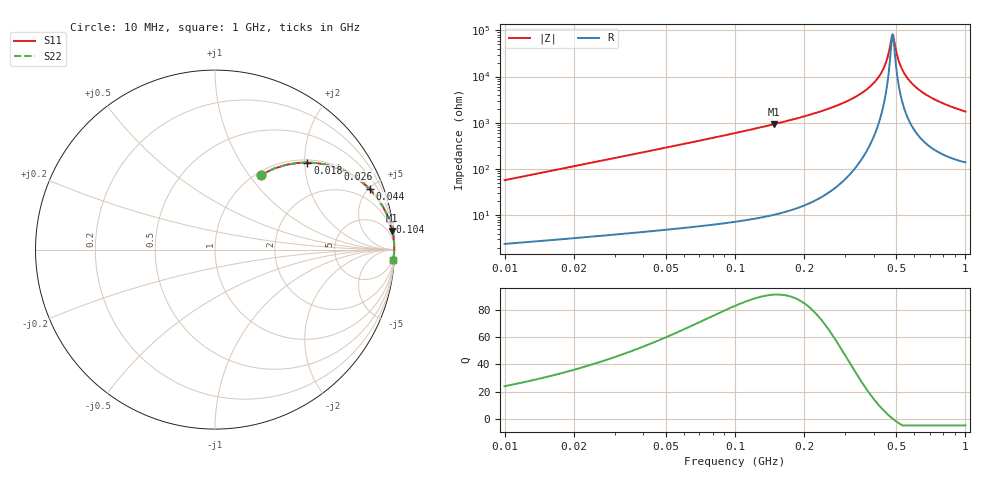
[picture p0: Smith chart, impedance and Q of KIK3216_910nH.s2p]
!version-2
!date-01.2022
!Series
# MHz S RI R 50
!Freq ReS11 ImS11 ReS21 ImS21 ReS12 ImS12 ReS22 ImS22
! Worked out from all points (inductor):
!   496 points, 10 MHz to 1 GHz, reference 50 ohm
!   read as one part in series: L = 910 nH near 14 MHz
!   highest Q = 91.3 at 148 MHz (marker M1), where L = 1 uH
!   self-resonance near 482 MHz
!   S11 on the Smith chart (normalised r, x): 10 MHz: 1.05, +1.14; 18 MHz: 1.06, +2.06; 26 MHz: 1.07, +2.98; 44 MHz: 1.09, +5.07; 104 MHz: 1, +12; 1 GHz: 4, -35
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10  0.2557 0.4158  0.7443 -0.4158  0.7443 -0.4158  0.2557 0.4158
18  0.5149 0.4852  0.4851 -0.4852  0.4851 -0.4852  0.5149 0.4852
26  0.6857 0.4524  0.3143 -0.4524  0.3143 -0.4524  0.6857 0.4524
44  0.8611 0.337  0.1389 -0.337  0.1389 -0.337  0.8611 0.337
66  0.9336 0.2418  0.0664 -0.2418  0.0664 -0.2418  0.9336 0.2418
104  0.9732 0.1558  0.0268 -0.1558  0.0268 -0.1558  0.9732 0.1558
148  0.9875 0.1056  0.0125 -0.1056  0.0125 -0.1056  0.9875 0.1056
176  0.9917 0.0854  0.00831 -0.0854  0.00831 -0.0854  0.9917 0.0854
340  0.9985 0.0259  0.00149 -0.0259  0.00149 -0.0259  0.9985 0.0259
396  0.9989 0.0145  0.00115 -0.0145  0.00115 -0.0145  0.9989 0.0145
434  0.9989 0.00779  0.00111 -0.00779  0.00111 -0.00779  0.9989 0.00779
458  0.9989 0.0039  0.00114 -0.0039  0.00114 -0.0039  0.9989 0.0039
478  0.9988 0.00081  0.0012 -0.00081  0.0012 -0.00081  0.9988 0.00081
482  0.9988 0.000209  0.00122 -0.000209  0.00122 -0.000209  0.9988 0.000209
488  0.9988 -0.000683  0.00124 0.000683  0.00124 0.000683  0.9988 -0.000683
506  0.9987 -0.0033  0.00132 0.0033  0.00132 0.0033  0.9987 -0.0033
528  0.9986 -0.00637  0.00144 0.00637  0.00144 0.00637  0.9986 -0.00637
562  0.9983 -0.0109  0.00167 0.0109  0.00167 0.0109  0.9983 -0.0109
608  0.9979 -0.0167  0.00206 0.0167  0.00206 0.0167  0.9979 -0.0167
670  0.9973 -0.0239  0.00269 0.0239  0.00269 0.0239  0.9973 -0.0239
836  0.9951 -0.0412  0.00492 0.0412  0.00492 0.0412  0.9951 -0.0412
1000  0.9922 -0.0564  0.00775 0.0564  0.00775 0.0564  0.9922 -0.0564
